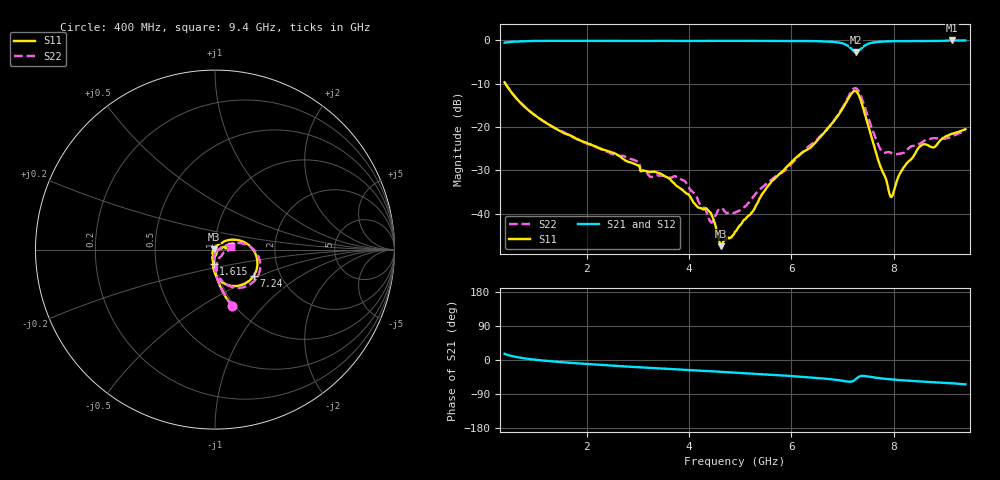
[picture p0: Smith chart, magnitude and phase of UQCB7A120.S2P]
!  Part Number  UQCB7A120	Mounting Orientation: Vertical
!  Description: RF capacitors
!  Application: Coupling, Bypass, Tuning, DC Block
!  Filters, Matching
# GHZ S DB R 50
! Freq  |S11|  S11 Ph  |S21|  S21 Ph  |S12|  S12 Ph  |S22|  S22 Ph
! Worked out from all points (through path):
!   401 points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, 400 MHz to 9.4 GHz, reference 50 ohm
!   highest |S21| = -0.01 dB at 9.13 GHz (marker M1); lowest = -2.7 dB at 7.263 GHz (marker M2)
!   group delay of S21, straight-line fit = 21.1 ps
!   lowest |S11| = -47.5 dB at 4.63 GHz (marker M3), VSWR 1.01, Z = 49.6 + j0.105 ohm
!   |S11| at or under -10 dB: 415.7 MHz to end of sweep
!   |S22| runs from -42.1 to -9.7 dB; largest |S21 - S12| = 0.0022
!   S11 on the Smith chart (normalised r, x): 400 MHz: 0.97, -0.68; 1.615 GHz: 0.97, -0.16; 7.24 GHz: 1.46, -0.46; 9.4 GHz: 1.20, +0.05
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0.4  -9.70 -73.3  -0.53 16.2  -0.52 16.2  -9.68 -72.9
0.895  -16.41 -86.8  -0.15 2.3  -0.14 2.3  -16.39 -85.6
1.615  -21.67 -95.3  -0.09 -6.8  -0.09 -6.8  -21.61 -93.0
1.908  -23.29 -99.3  -0.09 -9.6  -0.08 -9.6  -23.33 -93.8
3.415  -30.63 -114.3  -0.11 -22.1  -0.10 -22.1  -31.22 -92.8
3.91  -34.99 -137.4  -0.14 -26.0  -0.13 -26.0  -32.40 -106.9
4.383  -39.32 -165.4  -0.14 -29.4  -0.13 -29.4  -41.03 -96.0
4.63  -47.54 165.4  -0.10 -31.4  -0.10 -31.4  -38.73 -59.9
4.9  -44.23 117.7  -0.11 -33.5  -0.10 -33.5  -39.81 -36.4
5.62  -32.50 66.8  -0.14 -39.2  -0.14 -39.3  -32.12 7.6
6.408  -24.40 42.7  -0.17 -46.2  -0.17 -46.3  -23.87 20.4
7.015  -15.45 14.0  -0.74 -55.2  -0.75 -55.3  -15.19 9.4
7.24  -11.67 -34.5  -2.66 -52.5  -2.66 -52.6  -11.02 -32.0
7.263  -11.74 -42.3  -2.75 -50.0  -2.75 -50.1  -11.04 -39.0
7.443  -17.23 -89.2  -1.12 -42.4  -1.12 -42.5  -15.73 -79.8
7.735  -28.97 -86.8  -0.31 -48.2  -0.31 -48.3  -25.04 -70.1
7.915  -35.37 -56.8  -0.19 -50.7  -0.19 -50.8  -25.81 -45.4
7.983  -35.64 -19.6  -0.18 -51.7  -0.18 -51.8  -26.14 -40.0
8.14  -30.40 5.9  -0.18 -53.3  -0.19 -53.4  -26.12 -25.1
8.523  -24.39 13.2  -0.17 -56.8  -0.17 -56.9  -23.78 -6.2
9.13  -21.60 14.2  -0.01 -61.2  -0.01 -61.3  -22.17 5.8
9.4  -20.52 13.4  -0.01 -64.2  -0.01 -64.3  -20.88 10.8
